| TEXAS INSTRUMENTS INCORPORATED
| Standard Linear and Logic Group
| IBIS Model of SN74AUCH16244
| 16-BIT BUFFER/DRIVER WITH 3-STATE OUTPUTS
| This file contains package information for the following:
|  TSSOP 48-pin (DGG) package as [Component] AUCH16244_DGG
|  TVSOP 48-pin (DGV) package as [Component] AUCH16244_DGV
|  VFBGA 48-pin (GQL) package as [Component] AUCH16244_GQL
| This device can be powered at the following Vccs:
|  2.5 volt Vcc
|  1.8 volt Vcc
|  1.5 volt Vcc
|  1.2 volt Vcc
|  0.8 volt Vcc
| This file provides unique models under the [Model Selector] for each Vcc.
| For operation at a specific Vcc, select the appropriate model after each
| [Model Selector] keyword.
[IBIS Ver]   3.2
[Comment char]  |_char
[File Name]   sn74auch16244.ibs
[File Rev]   1.1 | x_die
[Date]   June 1, 2002
[Source]   Data created from TI-SPICE simulations at TI-SLL.
[Notes]   The following is an IBIS list for the SN74AUCH16244.
   Please contact sllibis@ti.com with questions and
   comments concerning SLL IBIS models.
   - The waveforms for the AUCH16244_OUT Power Clamp, Pullup,
   and Pulldown are caused by the circuitry that helps reduce
   overshoot and undershoot in transmission lines (EMI).
   These waveforms are normal for this particular design.
   - Due to presence of bus hold at input, GND-clamp curves
   have non-monotonic warnings.
[Disclaimer] Property of Texas Instruments Incorporated.  Unauthorized
   reproduction and/or distribution is strictly prohibited.
   This product is protected under copyright law.
   Created  2002, (C) Copyright  2002, Texas Instruments
   Incorporated, All Rights Reserved
   UNLESS THERE IS A SIGNED, WRITTEN AGREEMENT TO THE
   CONTRARY, TEXAS INSTRUMENTS (TI) IS PROVIDING THE IBIS
   MODELS  AND WITHOUT ANY WARRANTY, EXPRESSED OR
   IMPLIED.  TI assumes no liability for:
   1) the accuracy of the IBIS models provided to your
   company;
   2) the proper functioning of these IBIS Models in your
   design or for any resulting applications; or
   3) infringement of patents, copyrights or intellectual
   property rights resulting from your use of these IBIS
   models.
   TI provides IBIS Models as a service to our customers.
   You and your company shall not distribute, sell or give
   these models to anyone else without prior written
   permission from TI.
   TI reserves the right to make changes to our products or
   to discontinue any semiconductor product or service
   without notice, and advises our customers to obtain the
   latest version of relevant information to verify, before
   placing orders, that the information being relied on is
   current.
   Please be aware that your receipt and use of the IBIS
   information provided shall serve as acceptance of these
   terms and conditions.  If you do not accept these terms,
   you should return or destroy the IBIS models and any
   other accompanying information immediately.
| Component AUCH16244_DGG 48-pin TSSOP
[Component]   AUCH16244_DGG
[Manufacturer]  Texas Instruments, Inc.
[Package]
|   typ   min   max
R_pkg   6.200e-02   5.000e-02   7.800e-02
L_pkg   3.527e-09   3.128e-09   4.255e-09
C_pkg   5.300e-13   4.170e-13   6.850e-13
[Pin]   signal_name   model_name   R_pin   L_pin   C_pin
1   1NOE   AUCH16244_OE   5.000e-02   4.250e-09   6.710e-13
2   1Y1   AUCH16244_OUT   5.700e-02   3.956e-09   6.740e-13
3   1Y2   AUCH16244_OUT   7.100e-02   3.922e-09   6.190e-13
4   GND   GND   7.800e-02   3.841e-09   6.180e-13
5   1Y3   AUCH16244_OUT   5.600e-02   3.535e-09   5.550e-13
6   1Y4   AUCH16244_OUT   5.800e-02   3.464e-09   5.030e-13
7   VCC   POWER   6.000e-02   3.362e-09   4.980e-13
8   2Y1   AUCH16244_OUT   6.100e-02   3.293e-09   4.620e-13
9   2Y2   AUCH16244_OUT   6.300e-02   3.240e-09   4.550e-13
10   GND   GND   6.300e-02   3.175e-09   4.420e-13
11   2Y3   AUCH16244_OUT   6.400e-02   3.153e-09   4.290e-13
12   2Y4   AUCH16244_OUT   6.500e-02   3.128e-09   4.180e-13
13   3Y1   AUCH16244_OUT   6.500e-02   3.128e-09   4.180e-13
14   3Y2   AUCH16244_OUT   6.400e-02   3.154e-09   4.290e-13
15   GND   GND   6.300e-02   3.174e-09   4.420e-13
16   3Y3   AUCH16244_OUT   6.300e-02   3.241e-09   4.550e-13
17   3Y4   AUCH16244_OUT   6.100e-02   3.293e-09   4.620e-13
18   VCC   POWER   6.000e-02   3.362e-09   4.970e-13
19   4Y1   AUCH16244_OUT   5.800e-02   3.464e-09   5.030e-13
20   4Y2   AUCH16244_OUT   5.600e-02   3.537e-09   5.600e-13
21   GND   GND   7.700e-02   3.839e-09   6.260e-13
22   4Y3   AUCH16244_OUT   7.100e-02   3.917e-09   6.270e-13
23   4Y4   AUCH16244_OUT   5.800e-02   3.955e-09   6.850e-13
24   4NOE   AUCH16244_OE   5.200e-02   4.255e-09   6.790e-13
25   3NOE   AUCH16244_OE   5.100e-02   4.254e-09   6.760e-13
26   4A4   AUCH16244_IN   5.800e-02   3.957e-09   6.790e-13
27   4A3   AUCH16244_IN   7.100e-02   3.920e-09   6.210e-13
28   GND   GND   7.800e-02   3.843e-09   6.220e-13
29   4A2   AUCH16244_IN   5.600e-02   3.539e-09   5.600e-13
30   4A1   AUCH16244_IN   5.800e-02   3.466e-09   5.030e-13
31   VCC   POWER   6.000e-02   3.363e-09   4.970e-13
32   3A4   AUCH16244_IN   6.100e-02   3.294e-09   4.620e-13
33   3A3   AUCH16244_IN   6.300e-02   3.241e-09   4.540e-13
34   GND   GND   6.300e-02   3.175e-09   4.410e-13
35   3A2   AUCH16244_IN   6.400e-02   3.153e-09   4.290e-13
36   3A1   AUCH16244_IN   6.500e-02   3.129e-09   4.170e-13
37   2A4   AUCH16244_IN   6.500e-02   3.129e-09   4.170e-13
38   2A3   AUCH16244_IN   6.400e-02   3.152e-09   4.290e-13
39   GND   GND   6.400e-02   3.176e-09   4.410e-13
40   2A2   AUCH16244_IN   6.300e-02   3.241e-09   4.540e-13
41   2A1   AUCH16244_IN   6.100e-02   3.293e-09   4.620e-13
42   VCC   POWER   6.000e-02   3.363e-09   4.970e-13
43   1A4   AUCH16244_IN   5.800e-02   3.464e-09   5.030e-13
44   1A3   AUCH16244_IN   5.600e-02   3.534e-09   5.610e-13
45   GND   GND   7.800e-02   3.841e-09   6.260e-13
46   1A2   AUCH16244_IN   7.100e-02   3.920e-09   6.220e-13
47   1A1   AUCH16244_IN   5.700e-02   3.955e-09   6.770e-13
48   2NOE   AUCH16244_OE   5.100e-02   4.252e-09   6.720e-13
| Component AUCH16244_DGV 48-pin TVSOP
[Component]   AUCH16244_DGV
[Manufacturer]  Texas Instruments, Inc.
[Package]
|   typ   min   max
R_pkg   7.000e-02   4.900e-02   8.500e-02
L_pkg   3.013e-09   2.743e-09   3.408e-09
C_pkg   3.710e-13   2.940e-13   5.110e-13
[Pin]   signal_name   model_name   R_pin   L_pin   C_pin
1   1NOE   AUCH16244_OE   4.900e-02   3.393e-09   4.970e-13
2   1Y1   AUCH16244_OUT   6.000e-02   3.250e-09   5.020e-13
3   1Y2   AUCH16244_OUT   7.700e-02   3.310e-09   4.510e-13
4   GND   GND   8.500e-02   3.299e-09   4.040e-13
5   1Y3   AUCH16244_OUT   8.300e-02   3.136e-09   3.600e-13
6   1Y4   AUCH16244_OUT   7.700e-02   3.019e-09   3.630e-13
7   VCC   POWER   6.500e-02   2.882e-09   3.490e-13
8   2Y1   AUCH16244_OUT   6.600e-02   2.829e-09   3.140e-13
9   2Y2   AUCH16244_OUT   6.700e-02   2.796e-09   3.140e-13
10   GND   GND   6.900e-02   2.754e-09   3.080e-13
11   2Y3   AUCH16244_OUT   7.000e-02   2.753e-09   3.010e-13
12   2Y4   AUCH16244_OUT   7.100e-02   2.745e-09   2.940e-13
13   3Y1   AUCH16244_OUT   7.000e-02   2.744e-09   2.940e-13
14   3Y2   AUCH16244_OUT   7.000e-02   2.754e-09   3.010e-13
15   GND   GND   6.900e-02   2.754e-09   3.080e-13
16   3Y3   AUCH16244_OUT   6.700e-02   2.796e-09   3.140e-13
17   3Y4   AUCH16244_OUT   6.600e-02   2.829e-09   3.140e-13
18   VCC   POWER   6.500e-02   2.883e-09   3.500e-13
19   4Y1   AUCH16244_OUT   7.500e-02   3.014e-09   3.630e-13
20   4Y2   AUCH16244_OUT   8.000e-02   3.128e-09   3.580e-13
21   GND   GND   8.400e-02   3.295e-09   4.030e-13
22   4Y3   AUCH16244_OUT   7.800e-02   3.311e-09   4.520e-13
23   4Y4   AUCH16244_OUT   6.200e-02   3.259e-09   5.010e-13
24   4NOE   AUCH16244_OE   5.200e-02   3.404e-09   4.960e-13
25   3NOE   AUCH16244_OE   5.300e-02   3.397e-09   5.050e-13
26   4A4   AUCH16244_IN   6.200e-02   3.249e-09   5.110e-13
27   4A3   AUCH16244_IN   7.700e-02   3.308e-09   4.530e-13
28   GND   GND   8.200e-02   3.289e-09   4.030e-13
29   4A2   AUCH16244_IN   7.800e-02   3.121e-09   3.590e-13
30   4A1   AUCH16244_IN   7.400e-02   3.010e-09   3.630e-13
31   VCC   POWER   6.500e-02   2.883e-09   3.490e-13
32   3A4   AUCH16244_IN   6.700e-02   2.829e-09   3.140e-13
33   3A3   AUCH16244_IN   6.700e-02   2.795e-09   3.140e-13
34   GND   GND   6.900e-02   2.753e-09   3.070e-13
35   3A2   AUCH16244_IN   7.000e-02   2.753e-09   3.010e-13
36   3A1   AUCH16244_IN   7.000e-02   2.743e-09   2.940e-13
37   2A4   AUCH16244_IN   7.000e-02   2.743e-09   2.940e-13
38   2A3   AUCH16244_IN   7.000e-02   2.753e-09   3.010e-13
39   GND   GND   6.900e-02   2.754e-09   3.070e-13
40   2A2   AUCH16244_IN   6.800e-02   2.797e-09   3.140e-13
41   2A1   AUCH16244_IN   6.700e-02   2.830e-09   3.140e-13
42   VCC   POWER   6.400e-02   2.880e-09   3.490e-13
43   1A4   AUCH16244_IN   7.200e-02   3.004e-09   3.620e-13
44   1A3   AUCH16244_IN   7.800e-02   3.121e-09   3.590e-13
45   GND   GND   8.400e-02   3.296e-09   4.030e-13
46   1A2   AUCH16244_IN   7.700e-02   3.308e-09   4.510e-13
47   1A1   AUCH16244_IN   6.200e-02   3.258e-09   4.990e-13
48   2NOE   AUCH16244_OE   5.300e-02   3.408e-09   4.940e-13
| Component AUCH16244_GQL 48-pin VFBGA
[Component]   AUCH16244_GQL
[Manufacturer]  Texas Instruments, Inc.
[Package]
|   typ   min   max
R_pkg   7.900e-02   4.500e-02   9.400e-02
L_pkg   2.264e-09   1.398e-09   2.722e-09
C_pkg   3.060e-13   1.170e-13   4.040e-13
[Pin]   signal_name   model_name   R_pin   L_pin   C_pin
A1   1NOE   AUCH16244_OE   5.100e-02   1.531e-09   2.100e-13
B2   1Y1   AUCH16244_OUT   7.300e-02   2.572e-09   3.120e-13
B1   1Y2   AUCH16244_OUT   7.100e-02   1.835e-09   2.320e-13
B3   GND   GND   9.400e-02   2.717e-09   3.830e-13
C2   1Y3   AUCH16244_OUT   8.900e-02   2.534e-09   3.500e-13
C1   1Y4   AUCH16244_OUT   7.100e-02   1.831e-09   2.310e-13
C3   VCC   POWER   9.400e-02   2.722e-09   3.920e-13
D2   2Y1   AUCH16244_OUT   9.000e-02   2.551e-09   3.520e-13
D1   2Y2   AUCH16244_OUT   7.200e-02   1.846e-09   2.440e-13
D3   GND   GND   9.400e-02   2.719e-09   4.030e-13
E2   2Y3   AUCH16244_OUT   8.900e-02   2.541e-09   3.510e-13
E1   2Y4   AUCH16244_OUT   7.200e-02   1.850e-09   2.270e-13
F1   3Y1   AUCH16244_OUT   7.200e-02   1.850e-09   2.270e-13
F2   3Y2   AUCH16244_OUT   8.900e-02   2.541e-09   3.510e-13
G3   GND   GND   9.400e-02   2.718e-09   4.040e-13
G1   3Y3   AUCH16244_OUT   7.200e-02   1.847e-09   2.440e-13
G2   3Y4   AUCH16244_OUT   9.000e-02   2.551e-09   3.520e-13
H3   VCC   POWER   9.400e-02   2.721e-09   3.920e-13
H1   4Y1   AUCH16244_OUT   7.000e-02   1.830e-09   2.310e-13
H2   4Y2   AUCH16244_OUT   8.800e-02   2.524e-09   3.500e-13
J3   GND   GND   9.300e-02   2.709e-09   3.820e-13
J1   4Y3   AUCH16244_OUT   7.100e-02   1.851e-09   2.330e-13
J2   4Y4   AUCH16244_OUT   5.600e-02   2.605e-09   3.900e-13
K1   4NOE   AUCH16244_OE   4.500e-02   1.398e-09   1.170e-13
K6   3NOE   AUCH16244_OE   4.500e-02   1.512e-09   1.930e-13
J5   4A4   AUCH16244_IN   5.500e-02   2.492e-09   3.130e-13
J6   4A3   AUCH16244_IN   7.000e-02   1.821e-09   2.300e-13
J4   GND   GND   9.300e-02   2.703e-09   3.820e-13
H5   4A2   AUCH16244_IN   8.900e-02   2.529e-09   3.500e-13
H6   4A1   AUCH16244_IN   7.100e-02   1.826e-09   2.300e-13
H4   VCC   POWER   9.400e-02   2.722e-09   3.910e-13
G5   3A4   AUCH16244_IN   9.000e-02   2.551e-09   3.520e-13
G6   3A3   AUCH16244_IN   7.200e-02   1.846e-09   2.440e-13
G4   GND   GND   9.400e-02   2.719e-09   4.040e-13
F5   3A2   AUCH16244_IN   8.800e-02   2.510e-09   3.490e-13
F6   3A1   AUCH16244_IN   7.200e-02   1.850e-09   2.270e-13
E6   2A4   AUCH16244_IN   7.100e-02   1.850e-09   2.270e-13
E5   2A3   AUCH16244_IN   8.900e-02   2.529e-09   3.500e-13
D4   GND   GND   9.400e-02   2.719e-09   4.030e-13
D6   2A2   AUCH16244_IN   7.200e-02   1.847e-09   2.430e-13
D5   2A1   AUCH16244_IN   8.900e-02   2.550e-09   3.520e-13
C4   VCC   POWER   9.400e-02   2.722e-09   3.910e-13
C6   1A4   AUCH16244_IN   7.100e-02   1.827e-09   2.300e-13
C5   1A3   AUCH16244_IN   8.900e-02   2.539e-09   3.500e-13
B4   GND   GND   9.300e-02   2.705e-09   3.820e-13
B6   1A2   AUCH16244_IN   7.100e-02   1.831e-09   2.270e-13
B5   1A1   AUCH16244_IN   7.300e-02   2.685e-09   3.800e-13
A6   2NOE   AUCH16244_OE   5.100e-02   1.417e-09   1.330e-13
| Model AUCH16244_OE
[Model Selector]   AUCH16244_OE
AUCH16244_OE_25   2.5 volt Vcc
AUCH16244_OE_18   1.8 volt Vcc
AUCH16244_OE_15   1.5 volt Vcc
AUCH16244_OE_12   1.2 volt Vcc
AUCH16244_OE_08   0.8 volt Vcc
| Model AUCH16244_IN
[Model Selector]   AUCH16244_IN
AUCH16244_IN_25   2.5 volt Vcc
AUCH16244_IN_18   1.8 volt Vcc
AUCH16244_IN_15   1.5 volt Vcc
AUCH16244_IN_12   1.2 volt Vcc
AUCH16244_IN_08   0.8 volt Vcc
| Model AUCH16244_OUT
[Model Selector]   AUCH16244_OUT
AUCH16244_OUT_25   2.5 volt Vcc
AUCH16244_OUT_18   1.8 volt Vcc
AUCH16244_OUT_15   1.5 volt Vcc
AUCH16244_OUT_12   1.2 volt Vcc
AUCH16244_OUT_08   0.8 volt Vcc
| Models and submodels in the file (15): AUCH16244_OE_25 (Input), AUCH16244_OE_18 (Input), AUCH16244_OE_15 (Input), AUCH16244_OE_12 (Input), AUCH16244_OE_08 (Input), AUCH16244_IN_25 (Input), AUCH16244_IN_18 (Input), AUCH16244_IN_15 (Input), AUCH16244_IN_12 (Input), AUCH16244_IN_08 (Input), AUCH16244_OUT_25 (3-state), AUCH16244_OUT_18 (3-state), AUCH16244_OUT_15 (3-state), AUCH16244_OUT_12 (3-state), AUCH16244_OUT_08 (3-state)
